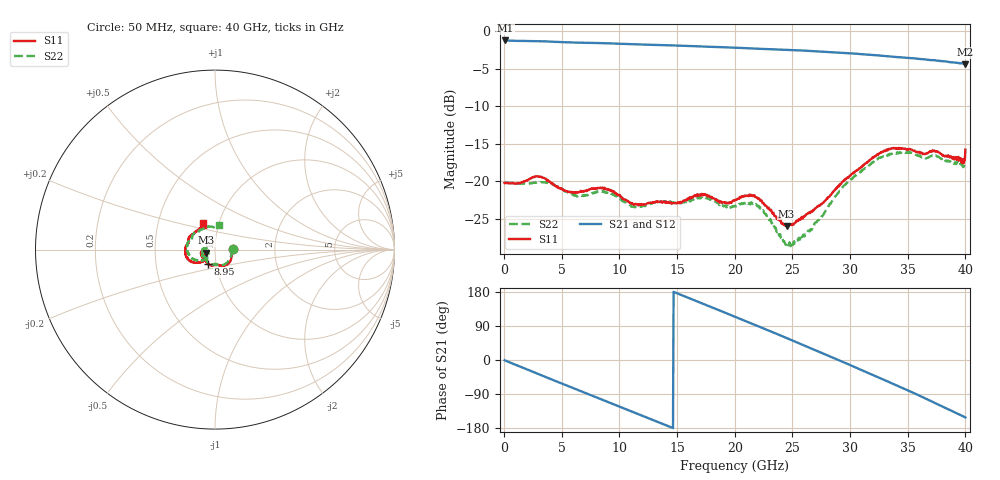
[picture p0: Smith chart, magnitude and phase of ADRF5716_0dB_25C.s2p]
! Device: ADRF5716
! Description: 30GHz 2-Bit Digital Attenuator
! Frequency: 100 MHz – 30 GHz
! Ports:
! ATTIN  = Port 1
! ATTOUT = Port 2
! State: 0 dB Attenuation selected
! Supply Voltage:
! VDD  =  +3.30 Volts
! VSS  =  -3.30 Volts
! Control Voltages:
! D5 = 0V, D6 = 0V
! Temperature = +25 C
! Data: Data was collected using a calibrated network analyzer.
!  The reference plane is the package pins of ADRF5716 switch.
! Note: Analog Devices supplies this data as a sample of measured data for this product.
!  Your particular data for this product may vary.
!  Analog Devices reserves the right to change this data at anytime
# HZ S DB R 50
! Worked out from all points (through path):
!   800 points, 50 MHz to 40 GHz, reference 50 ohm
!   highest |S21| = -1.23 dB at 100 MHz (marker M1); lowest = -4.4 dB at 40 GHz (marker M2)
!   group delay of S21, straight-line fit = 35.1 ps
!   lowest |S11| = -25.9 dB at 24.5 GHz (marker M3), VSWR 1.11, Z = 45.4 - j1.57 ohm
!   |S11| at or under -10 dB: start of sweep to end of sweep
!   |S22| runs from -28.6 to -16.1 dB; largest |S21 - S12| = 0
!   S11 on the Smith chart (normalised r, x): 50 MHz: 1.22, +0.00; 8.95 GHz: 0.91, -0.15; 40 GHz: 0.84, +0.26
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5e7  -20.21 0.6  -1.24 -0.6  -1.24 -0.6  -20.17 1.6
1e8  -20.18 -1.4  -1.23 -1.4  -1.23 -1.4  -20.15 -1.4
2e9  -19.91 -26.9  -1.30 -24.9  -1.30 -24.9  -20.31 -29.1
3.75e9  -19.79 -60.9  -1.37 -46.7  -1.37 -46.7  -20.21 -56.6
6.75e9  -21.34 -90.2  -1.54 -83.2  -1.54 -83.2  -21.95 -90.3
8.95e9  -21.03 -115.9  -1.61 -110.0  -1.61 -110.0  -21.49 -114.0
1.13e10  -23.08 -131.0  -1.75 -138.6  -1.75 -138.6  -23.44 -131.0
1.34e10  -22.71 -137.4  -1.84 -164.2  -1.84 -164.2  -22.63 -138.9
1.49e10  -22.90 -141.9  -1.91 177.3  -1.91 177.3  -22.84 -147.4
1.655e10  -21.91 -146.2  -2.00 157.3  -2.00 157.3  -22.33 -153.3
2.005e10  -22.43 -156.0  -2.20 113.7  -2.20 113.7  -23.24 -167.6
2.205e10  -22.34 -169.3  -2.33 88.9  -2.33 88.9  -23.27 179.1
2.45e10  -25.93 -160.1  -2.49 57.8  -2.49 57.8  -28.16 -171.6
2.67e10  -24.05 -141.7  -2.66 29.8  -2.66 29.8  -26.38 -141.5
2.83e10  -21.81 -135.5  -2.79 9.1  -2.79 9.1  -23.00 -136.0
2.99e10  -19.36 -138.9  -2.93 -11.9  -2.93 -11.9  -19.92 -142.7
3.15e10  -17.47 -147.2  -3.13 -33.3  -3.13 -33.3  -18.05 -153.4
3.335e10  -15.67 -164.7  -3.36 -57.8  -3.36 -57.8  -16.54 -172.5
3.495e10  -15.73 177.5  -3.55 -79.3  -3.55 -79.3  -16.12 169.1
3.645e10  -16.37 164.5  -3.76 -100.3  -3.76 -100.3  -16.84 154.1
3.805e10  -16.61 144.4  -3.99 -123.0  -3.99 -123.0  -17.19 133.8
4e10  -15.77 114.2  -4.42 -151.7  -4.42 -151.7  -17.27 80.7
